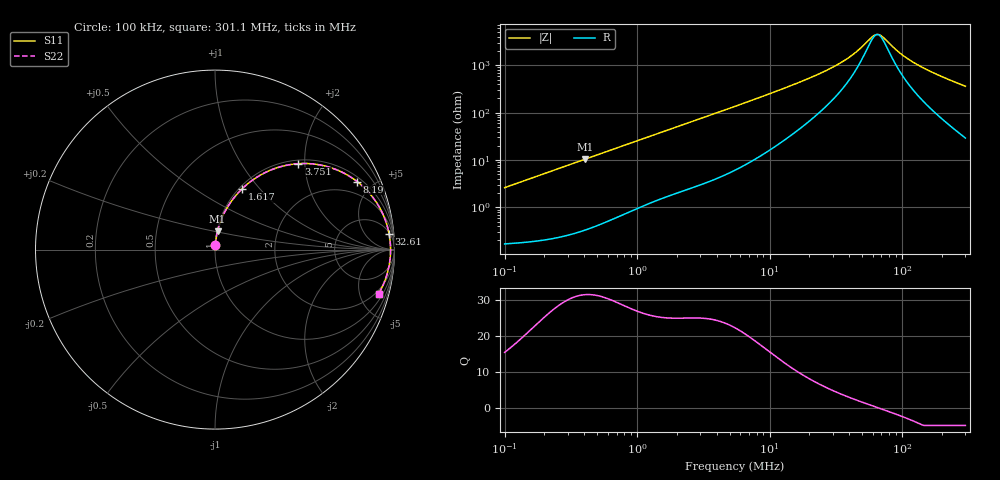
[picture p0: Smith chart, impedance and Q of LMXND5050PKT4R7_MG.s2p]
! LMXND5050PKT4R7_MG  S-PARAMETER MODEL  ( General Type )
! Model Generated by TAIYO YUDEN Corporation (http://www.ty-top.com)
! Version 1.0
! TAIYO YUDEN Control No. 191023NI43SB-FBB
! Copyright(c) 2019 TAIYO YUDEN CO.,LTD. All Rights Reserved.
! Product Description (link to TY-COMPAS)
! https://ds.yuden.co.jp/TYCOMPAS/or/detail?pn=LMXND5050PKT4R7NMG&u=M
! Products Name : Inductors
! Characteristics :
!  Inductance : 4.7 uH , SRF(min) : 41 MHz , DC Resistance(max) : 0.12 Ohm
!  Rated Current : Saturation :2050 mA , Temp Rise : 1400 mA
!  Case Size : 4.9 x 4.9 / 0.193 x 0.193 [mm/inch] , Thickness : 1.4 / 0.055 [mm/inch]
!  (Conditions: Temperature = 25 degC , DC Bias Current/Voltage = 0A / 0V)
! External Node Assignments :
!  1  o---GGG---o  2
! GND o---------o GND
! Frequency Range : 0.1MHz  -  301.082333MHz  [ 402 STEP ]
# MHz S RI R 50
! Freq[MHz].  S11 Real  S11 Imag  S21 Real  S21 Imag  S12 Real  S12 Imag  S22 Real  S22 Imag
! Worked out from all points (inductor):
!   401 points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, 100 kHz to 301.1 MHz, reference 50 ohm
!   read as one part in series: L = 4.12 uH near 104.1 kHz
!   highest Q = 31.5 at 406.2 kHz (marker M1), where L = 4.1 uH
!   self-resonance near 65.2 MHz
!   S11 on the Smith chart (normalised r, x): 100 kHz: 1.00, +0.05; 1.617 MHz: 1.03, +0.81; 3.751 MHz: 1.08, +1.85; 8.19 MHz: 1.23, +4.07; 32.61 MHz: 6, +20; 301.1 MHz: 1.58, -7.20
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0.1  0.00236 0.0259  0.9976 -0.0259  0.9976 -0.0259  0.00236 0.0259
0.382543  0.0126 0.0969  0.9874 -0.0969  0.9874 -0.0969  0.0126 0.0969
0.406228  0.014 0.1027  0.986 -0.1027  0.986 -0.1027  0.014 0.1027
0.852213  0.0517 0.2042  0.9483 -0.2042  0.9483 -0.2042  0.0517 0.2042
1.463388  0.1288 0.3158  0.8712 -0.3158  0.8712 -0.3158  0.1288 0.3158
1.617496  0.1511 0.3387  0.8489 -0.3387  0.8489 -0.3387  0.1511 0.3387
2.414223  0.2728 0.4258  0.7272 -0.4258  0.7272 -0.4258  0.2728 0.4258
3.750637  0.4636 0.4787  0.5364 -0.4787  0.5364 -0.4787  0.4636 0.4787
5.487097  0.6417 0.4576  0.3583 -0.4576  0.3583 -0.4576  0.6417 0.4576
8.189868  0.7929 0.3784  0.2071 -0.3784  0.2071 -0.3784  0.7929 0.3784
12.47119  0.8916 0.2745  0.1084 -0.2745  0.1084 -0.2745  0.8916 0.2745
20.99048  0.9499 0.162  0.0501 -0.162  0.0501 -0.162  0.9499 0.162
32.60995  0.9698 0.0891  0.0302 -0.0891  0.0302 -0.0891  0.9698 0.0891
43.16225  0.9754 0.0507  0.0246 -0.0507  0.0246 -0.0507  0.9754 0.0507
58.28473  0.978 0.0135  0.022 -0.0135  0.022 -0.0135  0.978 0.0135
63.14539  0.9782 0.00384  0.0218 -0.00384  0.0218 -0.00384  0.9782 0.00384
69.79514  0.9781 -0.00818  0.0219 0.00818  0.0219 0.00818  0.9781 -0.00818
80.29753  0.9776 -0.0251  0.0224 0.0251  0.0224 0.0251  0.9776 -0.0251
100.0843  0.9754 -0.0528  0.0246 0.0528  0.0246 0.0528  0.9754 -0.0528
132.4708  0.9696 -0.0915  0.0304 0.0915  0.0304 0.0915  0.9696 -0.0915
193.8017  0.9533 -0.1541  0.0467 0.1541  0.0467 0.1541  0.9533 -0.1541
301.0823  0.9118 -0.246  0.0882 0.246  0.0882 0.246  0.9118 -0.246
